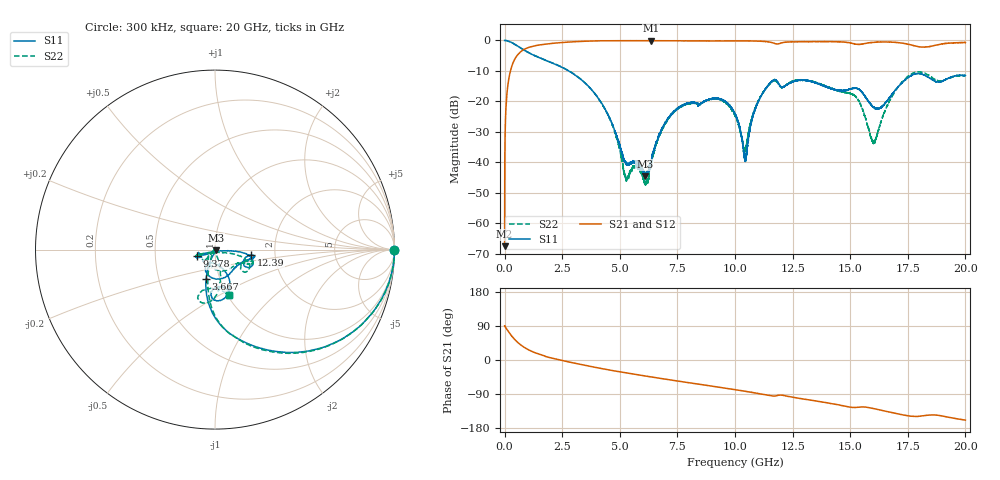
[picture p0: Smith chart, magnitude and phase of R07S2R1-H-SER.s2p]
!{R07S2R1}
!Johanson Technology Inc.
!www.johansontechnology.com
!Test Board Conditions:
!Substrate Type  RO4350B
!Substrate Thickness  10 mil
!Substrate Dk  3.66
!TL Type: GCPW
!TL Trace Width  21 mil
!TL Gap  20 mil
!Electrode orientation  Horizontal
!DUT TOPOLOGY	SERIES
!Mounting Pad LxW  16x21 mil
! Created Sat Feb  6 11:27:08 2021
# hz S ma R 50
! 2 Port Network Data from SP1.SP block
! freq  magS11  angS11  magS21  angS21  magS12  angS12  magS22  angS22
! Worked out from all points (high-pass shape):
!   20001 points, 300 kHz to 20 GHz, reference 50 ohm
!   highest |S21| = -0.07 dB at 6.36 GHz (marker M1); lowest = -67.5 dB at 300 kHz (marker M2)
!   |S21| within 3 dB of the highest: 819.2 MHz to end of sweep
!   lowest |S11| = -44.6 dB at 6.084 GHz (marker M3), VSWR 1.01, Z = 50.4 - j0.404 ohm
!   |S11| at or under -10 dB: 2.776 GHz to end of sweep
!   |S22| runs from -47.4 to 0.0 dB; largest |S21 - S12| = 0.012
!   S11 on the Smith chart (normalised r, x): 300 kHz: open; 3.667 GHz: 0.86, -0.29; 9.378 GHz: 0.81, -0.06; 12.39 GHz: 1.49, -0.10; 20 GHz: 1.02, -0.56
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300000  0.9999 -0.2  0.0004204 89.9  0.0003521 88.2  1 -0.2
1.253e8  0.9856 -11.1  0.1641 78.6  0.1648 78.5  0.9851 -11.2
4.443e8  0.8633 -35.5  0.4955 53.9  0.4969 53.9  0.8629 -35.7
3.3343e9  0.2258 -102.9  0.9647 -12.1  0.9657 -12.1  0.2275 -99.7
3.6673e9  0.1721 -106.9  0.9762 -16.2  0.9762 -16.2  0.1727 -103.4
4.6253e9  0.04704 -110.7  0.9897 -27.2  0.9901 -27.2  0.04503 -117.0
5.2573e9  0.009841 -58.8  0.9907 -33.9  0.9908 -33.9  0.005404 173.5
6.0843e9  0.005859 -43.1  0.9921 -42.0  0.9921 -42.1  0.004727 124.5
6.3603e9  0.01061 -113.5  0.9923 -44.7  0.9903 -44.7  0.009145 -151.2
6.6673e9  0.02583 -138.4  0.9898 -47.6  0.9896 -47.6  0.02477 -134.3
7.5743e9  0.07969 -158.3  0.9869 -56.1  0.9875 -56.1  0.07786 -132.6
9.3783e9  0.1083 -159.8  0.981 -72.5  0.9804 -72.4  0.1052 -163.2
1.00003e10  0.06157 -159.8  0.9829 -78.3  0.9822 -78.2  0.05828 -159.6
1.04493e10  0.01155 -80.2  0.9842 -82.7  0.9848 -82.6  0.01712 -77.5
1.12543e10  0.1449 -5.5  0.9626 -91.0  0.966 -90.8  0.1466 -14.6
1.23943e10  0.202 -8.8  0.9471 -97.3  0.9501 -97.2  0.2049 -17.2
1.33343e10  0.2109 -13.5  0.9547 -106.3  0.9552 -106.5  0.2133 -22.1
1.52343e10  0.165 -82.2  0.8697 -125.3  0.8698 -125.1  0.1212 -77.2
1.60033e10  0.08094 -113.5  0.9309 -128.0  0.9321 -128.0  0.02124 -115.5
1.66673e10  0.1097 -69.7  0.9444 -136.8  0.9335 -136.7  0.09535 -74.5
1.77903e10  0.2797 -80.9  0.8179 -149.0  0.8182 -148.6  0.2955 -97.0
2e10  0.2657 -73.0  0.9257 -158.7  0.9214 -158.8  0.2638 -72.5
